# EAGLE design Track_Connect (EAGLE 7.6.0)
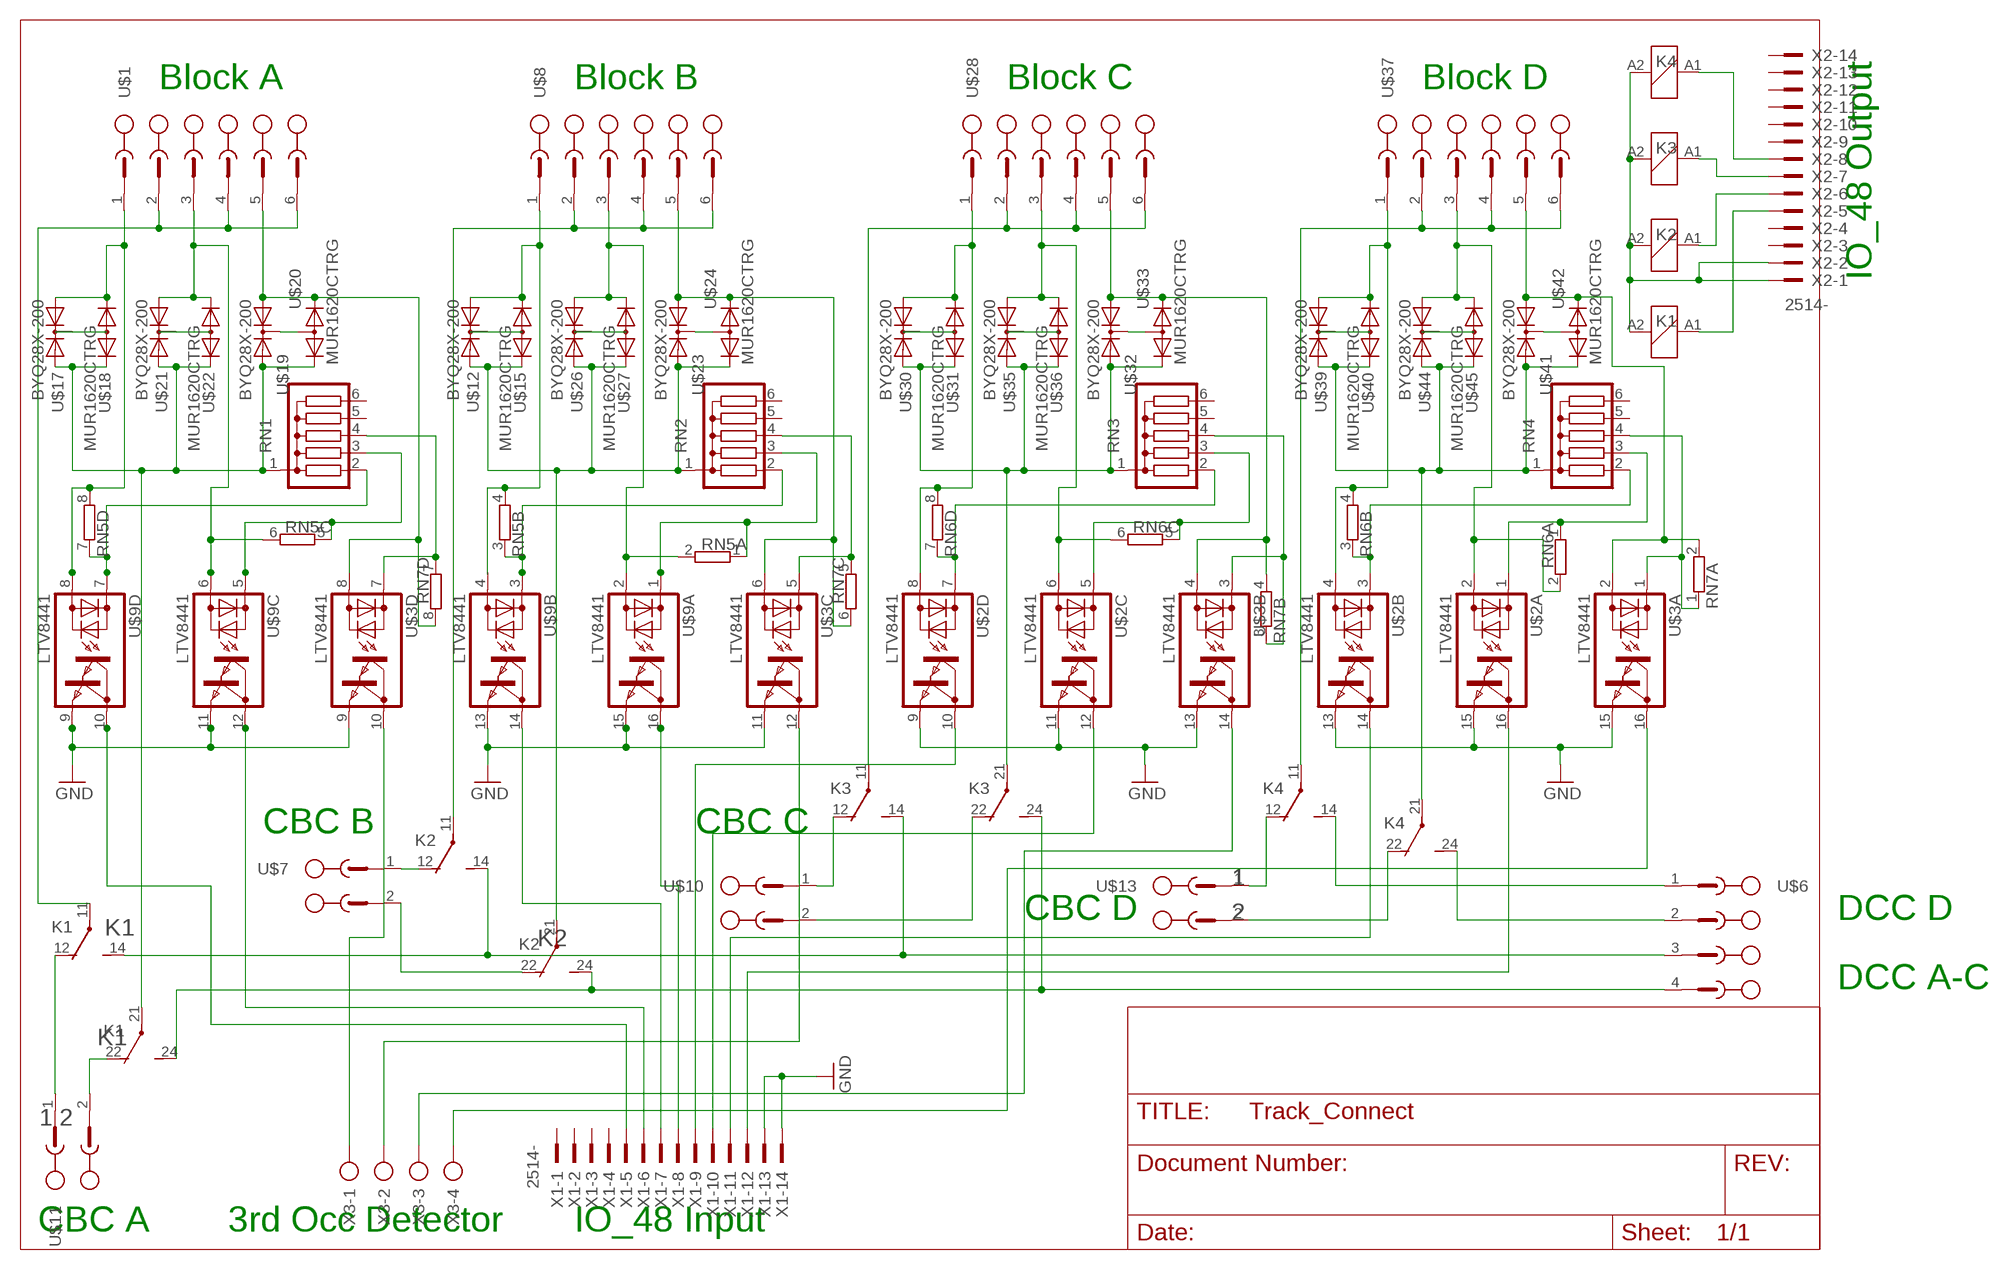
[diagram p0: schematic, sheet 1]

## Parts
K1  RT424012  [RT2C/O]
K2  RT424012  [RT2C/O]
K3  RT424012  [RT2C/O]
K4  RT424012  [RT2C/O]
RN1  G05R  [SIL6]
RN2  G05R  [SIL6]
RN3  G05R  [SIL6]
RN4  G05R  [SIL6]
RN5  E4R  [SIL8]
RN6  E4R  [SIL8]
RN7  E4R  [SIL8]
U$1  PT1_5_6-PVH-50  [PT1_5_6-PVH-50]
U$2  LTV8441  [DIL16]
U$3  LTV8441  [DIL16]
U$6  PT1_5_4-PVH-50  [PT1_5_4-PVH-50]
U$7  PT1_5_2-PVH-50  [PT1_5_2-PVH-50]
U$8  PT1_5_6-PVH-50  [PT1_5_6-PVH-50]
U$9  LTV8441  [DIL16]
U$10  PT1_5_2-PVH-50  [PT1_5_2-PVH-50]
U$11  PT1_5_2-PVH-50  [PT1_5_2-PVH-50]
U$12  BYQ28X-200  [TO220ABS]
U$13  PT1_5_2-PVH-50  [PT1_5_2-PVH-50]
U$15  MUR1620CTRG  [TO220ABS]
U$17  BYQ28X-200  [TO220ABS]
U$18  MUR1620CTRG  [TO220ABS]
U$19  BYQ28X-200  [TO220ABS]
U$20  MUR1620CTRG  [TO220ABS]
U$21  BYQ28X-200  [TO220ABS]
U$22  MUR1620CTRG  [TO220ABS]
U$23  BYQ28X-200  [TO220ABS]
U$24  MUR1620CTRG  [TO220ABS]
U$26  BYQ28X-200  [TO220ABS]
U$27  MUR1620CTRG  [TO220ABS]
U$28  PT1_5_6-PVH-50  [PT1_5_6-PVH-50]
U$30  BYQ28X-200  [TO220ABS]
U$31  MUR1620CTRG  [TO220ABS]
U$32  BYQ28X-200  [TO220ABS]
U$33  MUR1620CTRG  [TO220ABS]
U$35  BYQ28X-200  [TO220ABS]
U$36  MUR1620CTRG  [TO220ABS]
U$37  PT1_5_6-PVH-50  [PT1_5_6-PVH-50]
U$39  BYQ28X-200  [TO220ABS]
U$40  MUR1620CTRG  [TO220ABS]
U$41  BYQ28X-200  [TO220ABS]
U$42  MUR1620CTRG  [TO220ABS]
U$44  BYQ28X-200  [TO220ABS]
U$45  MUR1620CTRG  [TO220ABS]
X1  2514-  [PAK100/2500-14]
X2  2514-  [PAK100/2500-14]
X3  AK300/4  [AK300/4]

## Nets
GND: U$2.9(D:E) U$2.11(C:E) U$2.13(B:E) U$2.15(A:E) U$3.9(D:E) U$3.11(C:E) U$3.13(B:E) U$3.15(A:E) U$9.9(D:E) U$9.11(C:E) U$9.13(B:E) U$9.15(A:E) X1.13 X1.14
N$1: RN2.2 RN5.3 U$9.3(B:AC1)
N$2: RN1.3 RN5.5 U$9.5(C:AC1)
N$3 [Track]: K3.12(2:O) U$10.1(SK)
N$4: RN1.4 RN7.7 U$3.7(D:AC1)
N$5 [Track]: RN5.6 U$1.3(SK2) U$9.6(C:AC2) U$21.A1 U$22.A2(C2)
N$7 [Track]: U$21.C U$22.C(A)
N$8: RN2.3 RN5.1 U$9.1(A:AC1)
N$9: K1.21(3:P) RN1.1 U$17.A2 U$18.A1(C1) U$19.A2 U$20.A1(C1) U$21.A2 U$22.A1(C1)
N$12: K2.A1 X2.6
N$13 [Track]: K2.12(2:O) U$7.1(SK)
N$14 [Track]: K1.11(2:P) U$1.2(SK1) U$1.4(SK3) U$1.6(SK5)
N$15 [Track]: U$17.C U$18.C(A)
N$16 [Track]: K1.12(2:O) U$11.1(SK)
N$17 [Track]: K2.22(3:O) U$7.2(SK1)
N$18 [Track]: K1.22(3:O) U$11.2(SK1)
N$19: U$9.10(D:C1) X1.5
N$20 [Track]: RN7.2 U$3.2(A:AC2) U$37.5(SK4) U$41.A1 U$42.A2(C2)
N$21 [Track]: U$12.C U$15.C(A)
N$22: U$9.12(C:C1) X1.6
N$23 [Track]: RN5.8 U$1.1(SK) U$9.8(D:AC2) U$17.A1 U$18.A2(C2)
N$25 [Track]: U$19.C U$20.C(A)
N$26 [Track]: RN7.8 U$1.5(SK4) U$3.8(D:AC2) U$19.A1 U$20.A2(C2)
N$27 [Track]: U$23.C U$24.C(A)
N$28 [Track]: RN7.6 U$3.6(C:AC2) U$8.5(SK4) U$23.A1 U$24.A2(C2)
N$29: K2.21(3:P) RN2.1 U$12.A2 U$15.A1(C1) U$23.A2 U$24.A1(C1) U$26.A2 U$27.A1(C1)
N$30 [Track]: K2.11(2:P) U$8.2(SK1) U$8.4(SK3) U$8.6(SK5)
N$31 [Track]: U$26.C U$27.C(A)
N$32 [Track]: RN6.8 U$2.8(D:AC2) U$28.1(SK) U$30.A1 U$31.A2(C2)
N$33: RN2.4 RN7.5 U$3.5(C:AC1)
N$34: RN3.3 RN6.5 U$2.5(C:AC1)
N$35 [Track]: RN5.2 U$8.3(SK2) U$9.2(A:AC2) U$26.A1 U$27.A2(C2)
N$37 [Track]: RN5.4 U$8.1(SK) U$9.4(B:AC2) U$12.A1 U$15.A2(C2)
N$38: RN3.2 RN6.7 U$2.7(D:AC1)
N$39: RN1.2 RN5.7 U$9.7(D:AC1)
N$40: U$9.16(A:C1) X1.8
N$41: U$3.12(C:C1) X3.2
N$42: U$2.10(D:C1) X1.9
N$43 [Track]: K1.14(2:S) K2.14(2:S) K3.14(2:S) U$6.3(SK2)
N$44 [Track]: K1.24(3:S) K2.24(3:S) K3.24(3:S) U$6.4(SK3)
N$45: K1.A1 X2.5
N$46: K3.A1 X2.7
N$47 [Track]: U$30.C U$31.C(A)
N$49 [Track]: U$32.C U$33.C(A)
N$50 [Track]: RN7.4 U$3.4(B:AC2) U$28.5(SK4) U$32.A1 U$33.A2(C2)
N$51: K3.21(3:P) RN3.1 U$30.A2 U$31.A1(C1) U$32.A2 U$33.A1(C1) U$35.A2 U$36.A1(C1)
N$52 [Track]: K3.11(2:P) U$28.2(SK1) U$28.4(SK3) U$28.6(SK5)
N$53: U$2.12(C:C1) X1.10
N$54 [Track]: U$35.C U$36.C(A)
N$55 [Track]: RN6.6 U$2.6(C:AC2) U$28.3(SK2) U$35.A1 U$36.A2(C2)
N$56: RN3.4 RN7.3 U$3.3(B:AC1)
N$57: U$9.14(B:C1) X1.7
N$58: K1.A2 K2.A2 K3.A2 K4.A2 X2.1 X2.2
N$59: U$3.10(D:C1) X3.1
N$60 [Track]: K3.22(3:O) U$10.2(SK1)
N$62: RN4.2 RN6.3 U$2.3(B:AC1)
N$63: RN4.3 RN6.1 U$2.1(A:AC1)
N$64: U$2.14(B:C1) X1.11
N$65 [Track]: K4.12(2:O) U$13.1(SK)
N$67 [Track]: K4.11(2:P) U$37.2(SK1) U$37.4(SK3) U$37.6(SK5)
N$68 [Track]: U$39.C U$40.C(A)
N$69 [Track]: RN6.4 U$2.4(B:AC2) U$37.1(SK) U$39.A1 U$40.A2(C2)
N$70 [Track]: U$41.C U$42.C(A)
N$71: K4.A1 X2.8
N$73 [Track]: K4.21(3:P) RN4.1 U$39.A2 U$40.A1(C1) U$41.A2 U$42.A1(C1) U$44.A2 U$45.A1(C1)
N$75 [Track]: U$44.C U$45.C(A)
N$76: U$2.16(A:C1) X1.12
N$77: U$3.16(A:C1) X3.4
N$79 [Track]: K4.14(2:S) U$6.1(SK)
N$80 [Track]: K4.22(3:O) U$13.2(SK1)
N$81 [Track]: K4.24(3:S) U$6.2(SK1)
N$86: U$3.14(B:C1) X3.3
N$87 [Track]: RN6.2 U$2.2(A:AC2) U$37.3(SK2) U$44.A1 U$45.A2(C2)
N$88: RN4.4 RN7.1 U$3.1(A:AC1)
Unconnected: RN1.5 RN1.6 RN2.5 RN2.6 RN3.5 RN3.6 RN4.5 RN4.6 X1.1 X1.2 X1.3 X1.4 X2.3 X2.4 X2.9 X2.10 X2.11 X2.12 X2.13 X2.14

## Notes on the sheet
- Block A | Block B | Block C | Block D
- IO_48 Output
- CBC B | CBC C
- 1 | 1
- 2
- K1 | CBC D | DCC D
- K2
- DCC A-C
- K1
- 1 2
- CBC A | 3rd Occ Detector | IO_48 Input

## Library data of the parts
K1-K4 = relay:RT42?*: Power PCB Relay SCHRACK 2 pole 8 A, DC and AC-coil Source: http://www.schrack.com/.. 5842.pdf; MPN: RT424012; OC_FARNELL: 1629053; OC_NEWARK: 03P2426
RN1-RN4 = resistor-sil:G05R: SIL RESISTOR; OC_FARNELL: unknown; OC_NEWARK: unknown
RN5-RN7 = resistor-sil:E4R: SIL RESISTOR; OC_FARNELL: unknown; OC_NEWARK: unknown
U$1 U$8 U$28 U$37 = BDL-Boards:PT1_5_6-PVH-50
U$2 U$3 U$9 = optocoupler:LTV8441: Quad AC Optocoupler with Darlington Output
U$6 = BDL-Boards:PT1_5_4-PVH-50
U$7 U$11 = BDL-Board:PT1_5_2-PVH-50
U$10 U$13 = BDL-Boards:PT1_5_2-PVH-50
U$12 U$17 U$19 U$21 U$23 U$26 U$30 U$32 U$35 U$39 U$41 U$44 = diode:BYQ28X-200: Fast Recovery Diode Pair Common Cathode 10 Amps
U$15 U$18 U$20 U$22 U$24 U$27 U$31 U$33 U$36 U$40 U$42 U$45 = diode:MUR1620CTRG: Fast Recovery Diode Halfbridge 16 Amps
X1 X2 = con-3m:2514-: 3M (TM) Pak 100 4-Wall Header Source: 3M; OC_FARNELL: unknown; OC_NEWARK: unknown
X3 = con-ptr500:AK300/4: CONNECTOR; OC_FARNELL: unknown; OC_NEWARK: unknown

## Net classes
0 default: width 0.762 mm, drill 0.508 mm, clearance 0.381 mm
1 GND: width 0.762 mm, drill 0.508 mm, clearance 0.381 mm
2 VCC1: width 1.27 mm, drill 0.508 mm, clearance 0.381 mm
3 VCC2: width 0.762 mm, drill 0.508 mm, clearance 0.381 mm
4 Track: width 2.032 mm, drill 0.508 mm, clearance 0.381 mm

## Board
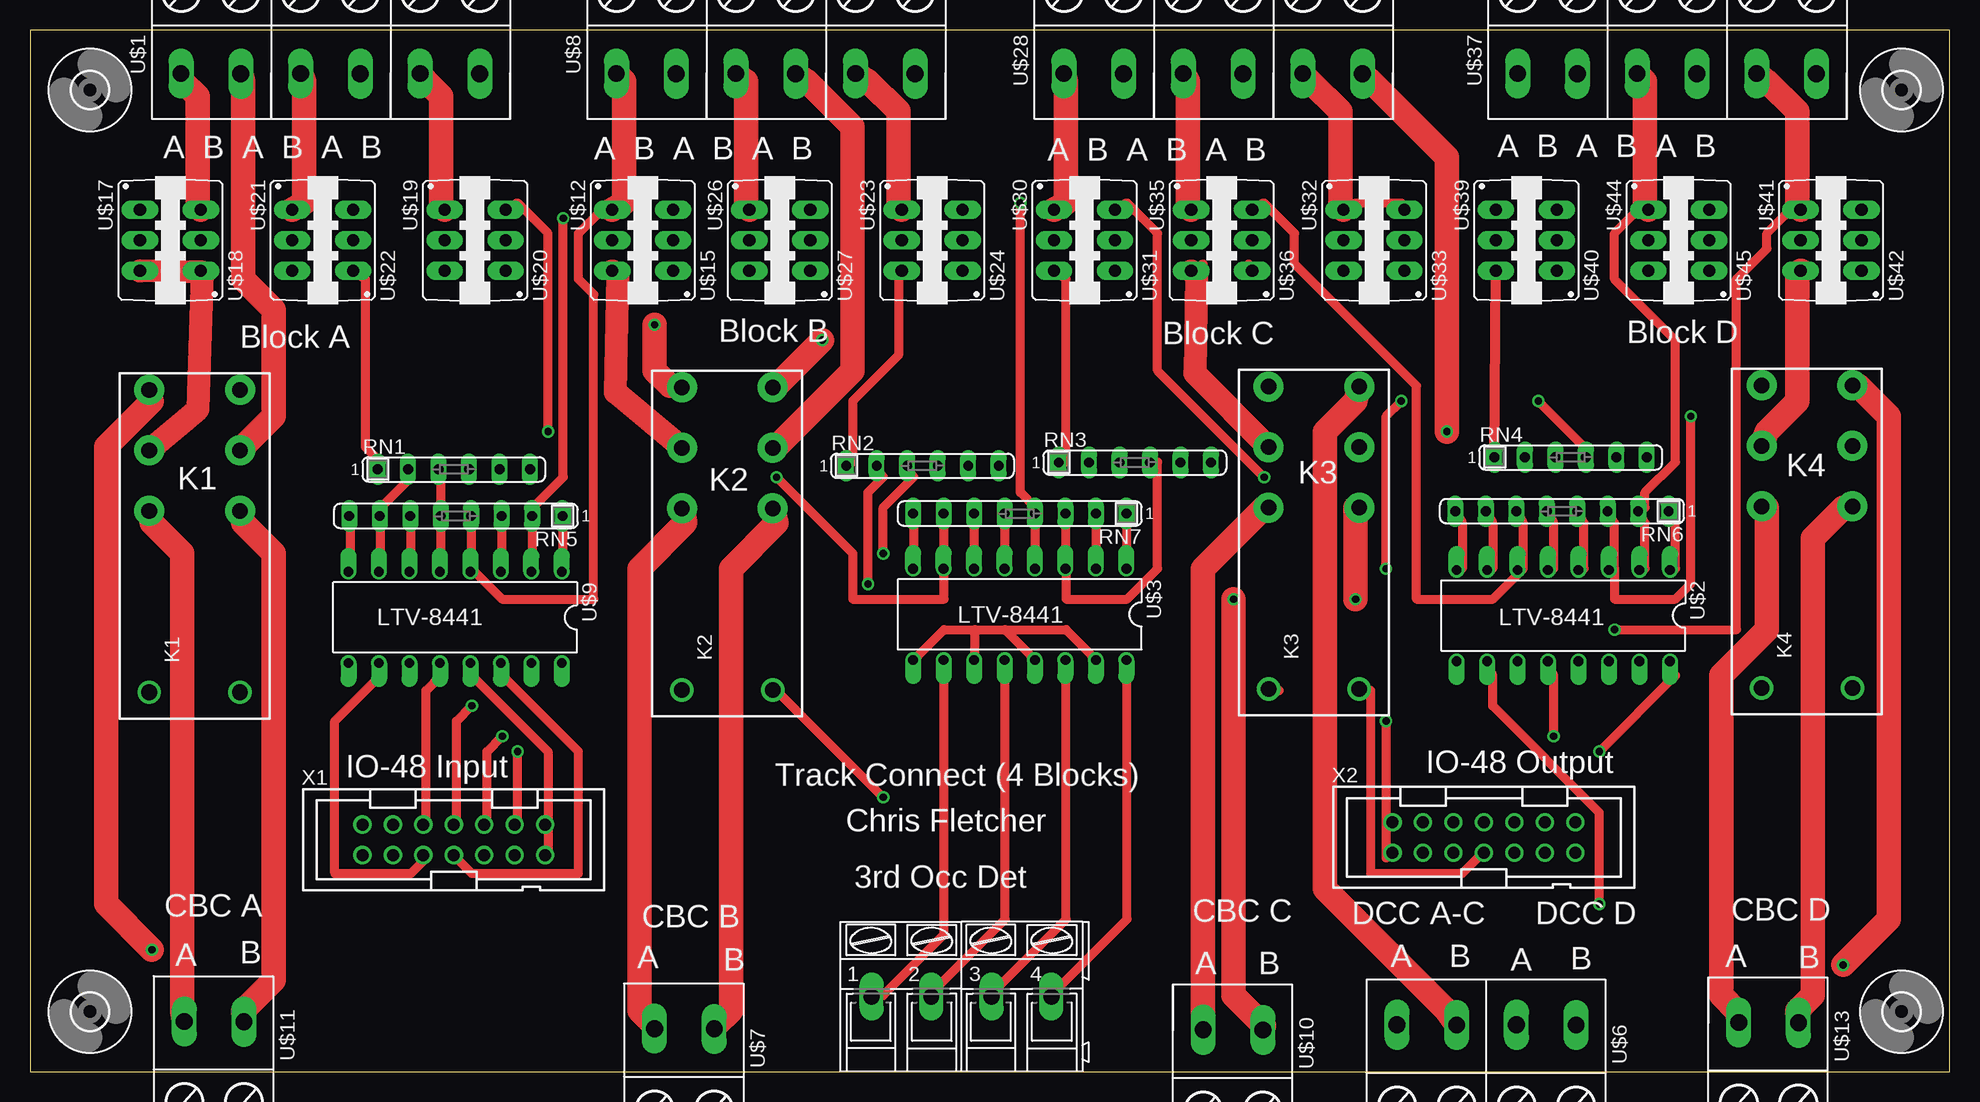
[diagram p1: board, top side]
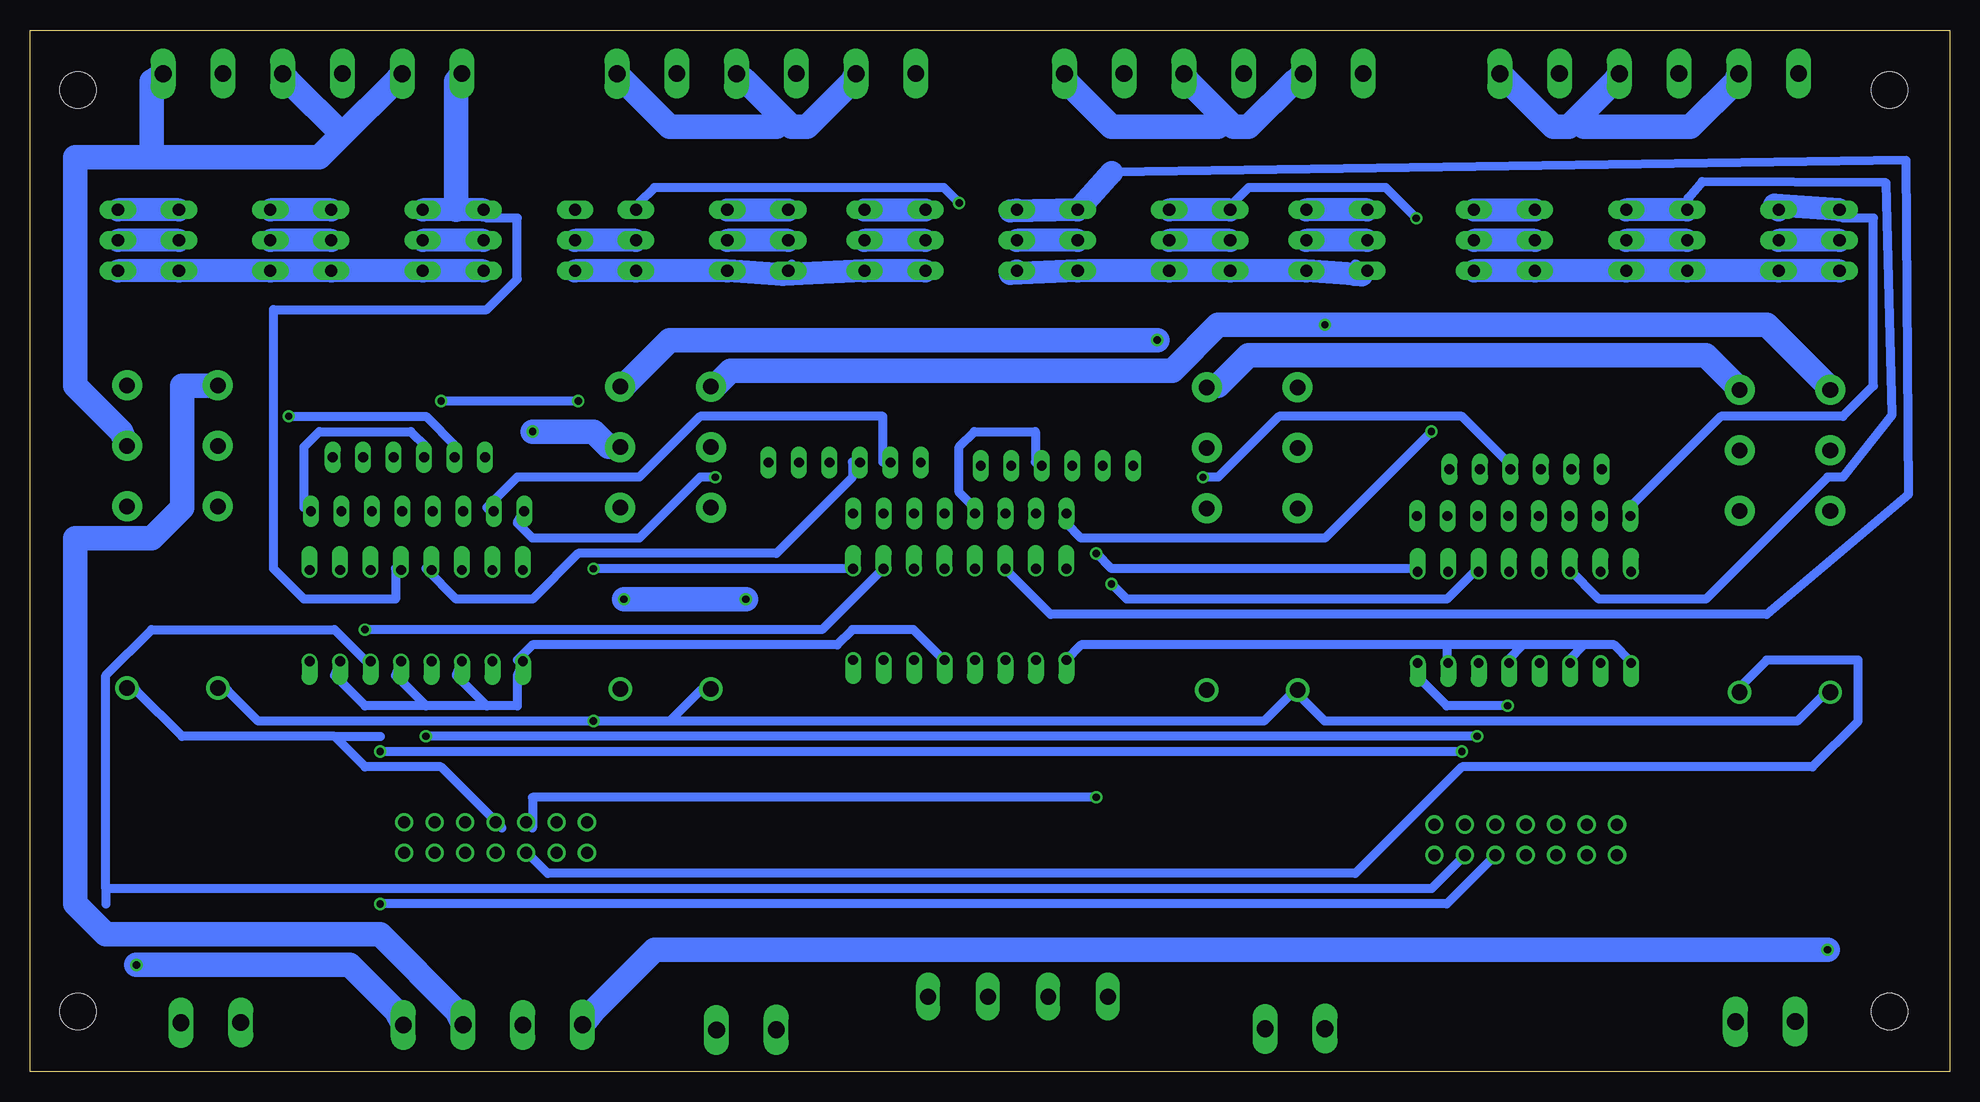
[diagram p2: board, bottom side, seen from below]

Size 160 x 86.8 mm. Coordinates in mm from the lower left corner, seen from the top.
Outline: 0,0 160,0 160,86.8 0,86.8 0,0
Copper layers (1*16): Top 0.035mm / dielectric 1.5mm / Bottom 0.035mm
Design rules "default": minimum track width 10mil, minimum drill 24mil, track to track 8mil, track to pad 8mil, pad to pad 8mil, via to via 8mil, smd to smd 8mil, copper to edge 40mil, drill to drill 8mil, minimum pad ring 10mil, minimum via ring 8mil, stop-mask expansion 4mil, vias tented up to drill 0mil, thermal gap 10mil

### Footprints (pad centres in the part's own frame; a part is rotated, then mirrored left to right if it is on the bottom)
3,0 = hole 3: 0,0
RT2C/O = drill 1.3 pad 2.5: 11 7.56,-3.68; 12 2.52,-3.68; 14 12.6,-3.68; 21 7.56,3.88; 22 2.52,3.88; 24 12.6,3.88 | drill 1.3: A1 -12.6,-3.68; A2 -12.6,3.88
SIL6 = drill 0.813 long: 1 -6.35,0; 2 -3.81,0; 3 -1.27,0; 4 1.27,0; 5 3.81,0; 6 6.35,0
SIL8 = drill 0.813 long: 1 -8.89,0; 2 -6.35,0; 3 -3.81,0; 4 -1.27,0; 5 1.27,0; 6 3.81,0; 7 6.35,0; 8 8.89,0
PT1_5_6-PVH-50 = drill 1.397 long: 1 17.157,2.42; 2 12.181,2.44; 3 7.197,2.42; 4 2.221,2.44; 5 -2.763,2.42; 6 -7.739,2.44
DIL16 = drill 0.813 offset: 1 -8.89,-3.81; 2 -6.35,-3.81; 3 -3.81,-3.81; 4 -1.27,-3.81; 5 1.27,-3.81; 6 3.81,-3.81; 7 6.35,-3.81; 8 8.89,-3.81; 9 8.89,3.81; 10 6.35,3.81; 11 3.81,3.81; 12 1.27,3.81; 13 -1.27,3.81; 14 -3.81,3.81; 15 -6.35,3.81; 16 -8.89,3.81
PT1_5_4-PVH-50 = drill 1.397 long: 1 4.457,6.23; 2 -0.519,6.25; 3 -5.503,6.23; 4 -10.479,6.25
PT1_5_2-PVH-50 = drill 1.397 long: 1 1.917,2.42; 2 -3.059,2.44
TO220ABS = drill 1.016 long: A1 -2.54,-2.54; A2 2.54,-2.54; C 0,-2.54
PAK100/2500-14 = drill 1 pad 1.422: 1 -7.62,-1.27; 2 -7.62,1.27; 3 -5.08,-1.27; 4 -5.08,1.27; 5 -2.54,-1.27; 6 -2.54,1.27; 7 0,-1.27; 8 0,1.27; 9 2.54,-1.27; 10 2.54,1.27; 11 5.08,-1.27; 12 5.08,1.27; 13 7.62,-1.27; 14 7.62,1.27
AK300/4 = drill 1.321 long: 1 -7.493,0; 2 -2.515,0; 3 2.515,0; 4 7.493,0

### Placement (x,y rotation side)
E$1  [3,0]  5,81.8 0 top
E$2  [3,0]  156,81.8 0 top
E$3  [3,0]  5,5 0 top
E$4  [3,0]  156,5 0 top
K1  13.82,44.21 90 top
K2  58.22,44.41 90 top
K3  107.12,44.48 90 top
K4  148.22,44.58 90 top
RN1  35.33,50.19 0 top
RN2  74.39,50.49 0 top
RN3  92.09,50.76 0 top
RN4  128.42,51.19 0 top
RN5  35.5,46.3 180 top
RN6  127.7,46.7 180 top
RN7  82.5,46.5 180 top
U$1  29.75,85.59 180 top
U$2  127.8,38 180 top
U$3  82.5,38.1 180 top
U$6  124.42,-2.34 0 top
U$7  55.12,1.14 0 top
U$8  66.04,85.59 180 top
U$9  35.44,37.85 180 top
U$10  100.86,1.05 0 top
U$11  15.92,1.74 0 top
U$12  51.07,69.27 270 top
U$13  145.49,1.65 0 top
U$15  51.07,69.27 90 top
U$17  11.7,69.27 270 top
U$18  11.7,69.27 90 top
U$19  37.1,69.27 270 top
U$20  37.1,69.27 90 top
U$21  24.4,69.27 270 top
U$22  24.4,69.27 90 top
U$23  75.2,69.27 270 top
U$24  75.2,69.27 90 top
U$26  62.5,69.27 270 top
U$27  62.5,69.27 90 top
U$28  103.33,85.59 180 top
U$30  87.9,69.27 270 top
U$31  87.9,69.27 90 top
U$32  112.03,69.27 270 top
U$33  112.03,69.27 90 top
U$35  99.33,69.27 270 top
U$36  99.33,69.27 90 top
U$37  141.16,85.59 180 top
U$39  124.73,69.27 270 top
U$40  124.73,69.27 90 top
U$41  150.13,69.27 270 top
U$42  150.13,69.27 90 top
U$44  137.43,69.27 270 top
U$45  137.43,69.27 90 top
X1  35.33,19.32 0 top
X2  121.2,19.52 0 top
X3  77.64,6.25 0 top

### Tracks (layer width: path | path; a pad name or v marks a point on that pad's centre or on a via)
GND
  Top 0.762: 78.74,36.83 76.2,36.83 73.66,34.29 U$3.9 | 78.74,36.83 78.74,34.29 U$3.11 | 81.28,36.83 83.82,34.29 U$3.13 | 78.74,36.83 81.28,36.83 | 81.28,36.83 86.36,36.83 88.9,34.29 U$3.15 | U$9.13 36.83,33.02 43.18,26.67 43.18,20.32 | 43.18,20.32 43.18,17.78 X1.13 | 43.18,20.32 X1.14
  Bottom 0.762: 121.92,30.48 119.38,30.48 119.38,33.02 U$2.9 119.38,34.29 118.11,35.56 92.71,35.56 91.44,36.83 86.36,36.83 83.82,34.29 U$3.13 | 121.92,30.48 124.46,33.02 U$2.11 | 127,30.48 129.54,33.02 U$2.13 | 121.92,30.48 127,30.48 | 127,30.48 132.08,30.48 134.62,33.02 U$2.15 | 30.48,35.56 27.94,35.56 26.67,34.29 U$9.9 | 30.48,35.56 31.75,34.29 U$9.11 | 35.56,35.56 36.83,34.29 U$9.13 | 30.48,35.56 35.56,35.56 | 35.56,35.56 41.91,35.56 | 41.91,35.56 72.39,35.56 73.66,34.29 U$3.9 | 41.91,35.56 41.91,34.29 U$9.15
N$1  (via drill 0.61)
  Top 0.762: U$9.3 39.37,41.91 39.37,45.72 RN5.3 | v69.85,40.64 69.85,48.26 71.12,49.53 RN2.2
  Bottom 0.762: v69.85,40.64 68.58,39.37 41.91,39.37 39.37,41.91 U$9.3
N$2
  Top 0.762: U$9.5 34.29,41.91 34.29,45.72 RN5.5 34.29,46.99 34.29,49.53 RN1.3
N$3  (via drill 0.61)
  Top 2.032: v100.33,39.37 100.33,6.35 102.87,3.81 U$10.1 | v110.49,39.37 110.49,46.99 K3.12
  Bottom 2.032: v100.33,39.37 v110.49,39.37
N$4  (via drill 0.61)
  Top 0.762: 76.2,41.91 76.2,45.72 RN7.7 | v62.23,49.53 68.58,43.18 68.58,39.37 76.2,39.37 76.2,41.91 | 76.2,41.91 U$3.7
  Bottom 0.762: v62.23,49.53 60.96,49.53 55.88,54.61 40.64,54.61 36.83,50.8 RN1.4
N$5
  Top 0.762: U$9.6 31.75,41.91 31.75,45.72 RN5.6
  Top 2.032: U$1.3 22.86,82.55 22.86,72.39 U$21.A1
  Bottom 0.762: U$9.6 31.75,41.91 29.21,39.37 20.32,39.37 10.16,49.53 8.89,49.53 4.78,54.74 5.28,74.06 20.62,74.16 21.79,72.79 U$21.A1
  Bottom 1.93: U$21.A1 U$22.A2
N$7
  Bottom 1.93: U$21.C U$22.C
N$8  (via drill 0.61)
  Top 0.762: U$9.1 44.45,41.91 44.45,45.72 RN5.1 | v71.12,43.18 71.12,46.99 73.66,49.53 RN2.3
  Bottom 0.762: v71.12,43.18 69.85,41.91 44.45,41.91 U$9.1
N$9
  Top 0.762: RN1.1 29.21,50.8 27.94,52.07 27.94,66.04 U$22.A1
  Top 1.93: U$17.A2 14.4,66.6 14,55.2 K1.21
  Bottom 1.93: U$17.A2 U$18.A1 U$21.A2 U$22.A1 U$19.A2 U$20.A1
N$12  (via drill 0.61)
  Top 0.762: v71.12,22.86 62.23,31.75 K2.A1
  Bottom 0.762: v71.12,22.86 118.11,22.86 118.11,20.32 X2.6
N$13
  Top 2.032: U$7.1 57.15,3.81 58.42,5.08 58.42,41.91 62.23,45.72 K2.12
N$14
  Top 2.032: K1.11 17.78,52.07 20.32,54.61 20.32,63.5 17.78,66.04 17.78,82.55 U$1.2
  Bottom 2.032: 31.11,79.38 31.75,78.74 33.02,78.74 36.83,82.55 U$1.6 | 31.11,79.38 27.94,82.55 U$1.4 | U$1.2 17.78,82.55 21.59,78.74 30.48,78.74 31.11,79.38
N$15
  Bottom 1.93: U$17.C U$18.C
N$16
  Top 2.032: U$11.1 17.78,5.08 20.32,7.62 20.32,43.18 17.78,45.72 K1.12
N$17
  Top 2.032: U$7.2 52.07,3.81 50.8,5.08 50.8,41.91 54.61,45.72 K2.22
N$18
  Top 2.032: U$11.2 12.7,5.08 12.7,43.18 10.16,45.72 K1.22
N$19
  Top 0.762: U$9.10 29.21,33.02 25.4,29.21 25.4,16.51 31.75,16.51 33.02,17.78 X1.5
N$20  (via drill 0.61)
  Top 0.762: U$3.2 88.9,41.91 88.9,45.72 RN7.2 | v132.08,36.83 142.24,36.83 142.24,66.04 144.78,68.58 144.78,69.85 147.32,72.39
  Top 2.032: U$37.5 144.78,82.55 147.32,80.01 147.32,72.39 U$41.A1
  Bottom 0.762: v132.08,36.83 93.98,36.83 88.9,41.91 U$3.2
  Bottom 1.93: U$41.A1 U$42.A2
N$21
  Bottom 1.93: U$12.C U$15.C
N$22
  Top 0.762: U$9.12 34.29,33.02 33.02,31.75 33.02,20.32 X1.6
N$23
  Top 0.762: U$9.8 26.67,41.91 26.67,45.72 RN5.8
  Top 2.032: U$1.1 12.7,82.55 13.97,81.28 13.97,72.39 U$18.A2
  Bottom 0.762: RN5.8 26.67,46.99 19.05,54.61 8.89,54.61 6.35,57.15 6.35,71.12 8.89,71.12 U$17.A1
  Bottom 1.93: U$17.A1 14.6,72.2 U$18.A2
N$25
  Bottom 1.93: U$19.C U$20.C
N$26  (via drill 0.61)
  Top 0.762: U$3.8 73.66,41.91 73.66,45.72 RN7.8 | v43.18,53.34 43.18,69.85 40.64,72.39 U$20.A2
  Top 2.032: U$1.5 33.02,82.55 34.29,81.28 34.29,72.39 U$19.A1
  Bottom 0.762: v43.18,53.34 52.07,44.45 72.39,44.45 73.66,45.72 RN7.8
  Bottom 1.93: U$20.A2 U$19.A1
N$27
  Bottom 1.93: U$23.C U$24.C
N$28
  Top 0.762: U$3.6 78.74,41.91 78.74,45.72 RN7.6
  Top 2.032: U$8.5 69.85,82.55 72.39,80.01 72.39,72.39 U$23.A1
  Bottom 0.762: U$3.6 78.74,41.91 74.93,38.1 15.24,38.1 3.41,48.13 3.61,75.93 69.85,74.93 72.39,72.39 U$23.A1
  Bottom 1.93: U$23.A1 78.3,71.7 U$24.A2 | 69.85,74.93 72.7,71.8
N$29
  Top 0.762: RN2.1 68.58,50.8 68.58,55.88 72.39,59.69 72.39,66.04 U$23.A2
  Top 1.93: K2.21 48.8,56.6 49,66.4 U$12.A2
  Bottom 0.762: U$12.A2 49.53,67.31 49.59,66.45
  Bottom 1.93: 49,66.4 49.59,66.45 U$15.A1 U$26.A2 U$27.A1 U$23.A2 78.3,66.5 U$24.A1
N$30
  Top 2.032: K2.11 62.23,52.07 68.58,58.42 68.58,78.74 64.77,82.55 U$8.4
  Bottom 2.032: 60.33,79.38 63.5,82.55 U$8.4 | 60.33,79.38 59.69,78.74 58.42,78.74 54.61,82.55 U$8.2 | U$8.6 73.66,82.55 69.85,78.74 60.96,78.74 60.33,79.38
N$31
  Bottom 1.93: U$26.C U$27.C
N$32  (via drill 0.61)
  Top 0.762: RN6.8 119.38,45.72 119.38,41.91 U$2.8 | v102.87,49.53 93.98,58.42 93.98,69.85 91.44,72.39 U$31.A2
  Top 2.032: U$28.1 86.36,82.55 86.36,72.39 U$30.A1
  Bottom 0.762: v102.87,49.53 104.14,49.53 109.22,44.45 118.11,44.45 119.38,45.72 RN6.8
  Bottom 1.93: U$31.A2 U$30.A1
N$33
  Top 0.762: U$3.5 81.28,41.91 81.28,45.72 RN7.5
  Bottom 0.762: RN2.4 76.2,50.8 76.2,53.34 81.28,53.34 82.55,52.07 82.55,48.26 81.28,46.99 RN7.5
N$34
  Top 0.762: RN6.5 127,45.72 127,41.91 U$2.5
  Bottom 0.762: RN3.3 91.44,50.8 91.44,49.53 97.79,43.18 114.3,43.18 118.11,39.37 124.46,39.37 127,41.91 U$2.5
N$35  (via drill 0.61)
  Top 0.762: U$9.2 41.91,41.91 41.91,45.72 RN5.2 41.91,46.99 44.45,49.53 v44.45,71.12
  Top 2.032: U$8.3 59.69,82.55 59.69,72.39 U$26.A1
  Bottom 0.762: v44.45,71.12 46.99,73.66 58.42,73.66 59.69,72.39 U$26.A1
  Bottom 1.93: U$26.A1 U$27.A2
N$37
  Top 0.762: 36.83,41.91 36.83,45.72 RN5.4 | 36.83,41.91 39.37,39.37 46.99,39.37 46.99,64.77 45.72,66.04 45.72,69.85 48.26,72.39 U$12.A1 | U$9.4 36.83,41.91
  Top 2.032: U$8.1 49.53,82.55 49.53,72.39 U$12.A1
  Bottom 1.93: U$12.A1 U$15.A2
N$38
  Top 0.762: RN6.7 121.92,45.72 121.92,41.91 U$2.7
  Bottom 0.762: RN3.2 88.9,50.8 88.9,54.61 104.14,54.61 109.22,49.53 119.38,49.53 121.92,46.99 RN6.7
N$39
  Top 0.762: U$9.7 29.21,41.91 29.21,45.72 RN5.7 29.21,46.99 31.75,49.53 RN1.2
N$40  (via drill 0.61)
  Top 0.762: v36.83,30.48 35.56,29.21 35.56,20.32 X1.8
  Bottom 0.762: v36.83,30.48 41.91,30.48 44.45,33.02 U$9.16
N$41
  Top 0.762: U$3.12 81.28,34.29 81.28,12.7 74.93,6.35 X3.2
N$42  (via drill 0.61)
  Top 0.762: v130.81,13.97 130.81,21.59 121.92,30.48 121.92,33.02 U$2.10
  Bottom 0.762: v130.81,13.97 41.91,13.97 38.1,17.78 X1.9
N$43  (via drill 0.61)
  Top 2.032: K3.14 110.49,55.88 107.95,53.34 107.95,15.24 118.11,5.08 U$6.3 | v66.04,60.96 62.23,57.15 K2.14
  Bottom 2.032: K1.14 17.78,57.15 20.32,59.69 58.42,59.69 60.96,57.15 K2.14 | v66.04,60.96 106.68,60.96 110.49,57.15 K3.14
N$44  (via drill 0.61)
  Top 2.032: v10.16,10.16 6.35,13.97 6.35,52.07 10.16,55.88 K1.24 | v52.07,62.23 52.07,58.42 53.34,57.15 K2.24
  Bottom 2.032: v10.16,10.16 107.95,10.16 113.03,5.08 U$6.4 | K1.24 10.16,57.15 15.24,62.23 v52.07,62.23 60.96,62.23 64.77,58.42 101.6,58.42 102.87,57.15 K3.24
N$45
  Bottom 0.762: K1.A1 17.78,31.75 15.24,34.29 7.62,34.29 7.62,29.21 11.43,25.4 40.64,25.4 49.53,16.51 116.84,16.51 118.11,17.78 X2.5
N$46
  Top 0.762: 110.49,31.75 K3.A1 111.76,31.75 111.76,16.51 119.38,16.51 120.65,17.78 X2.7
N$47
  Bottom 1.93: U$30.C U$31.C
N$49
  Bottom 1.93: U$32.C U$33.C
N$50  (via drill 0.61)
  Top 0.762: U$3.4 83.82,41.91 83.82,45.72 RN7.4 83.82,46.99 82.55,48.26 v82.55,72.39 | U$33.A2 114.3,72.39 110.49,72.39 U$32.A1
  Top 2.032: U$28.5 106.68,82.55 109.22,80.01 109.22,72.39 U$32.A1
  Bottom 0.762: v82.55,72.39 83.82,73.66 107.95,73.66 109.22,72.39 U$32.A1
N$51
  Top 0.762: U$35.A2 97.79,67.31 | U$36.A1 101.6,67.31 | RN3.1 86.36,50.8 86.36,66.04 U$30.A2
  Top 1.93: K3.21 97.1,58.2 97.24,66.42 U$35.A2
  Bottom 0.762: 96.48,66.45 96.52,67.31 U$35.A2
  Bottom 1.93: U$33.A1 U$32.A2 U$36.A1 97.24,66.42 96.48,66.45 U$31.A1 U$30.A2
N$52  (via drill 0.61)
  Top 2.032: v118.11,53.34 118.11,76.2 111.76,82.55 U$28.6
  Bottom 2.032: 97.16,79.38 100.33,82.55 U$28.4 | 97.16,79.38 96.52,78.74 95.25,78.74 91.44,82.55 U$28.2 | U$28.6 110.49,82.55 106.68,78.74 97.79,78.74 97.16,79.38 | v118.11,53.34 113.03,53.34 111.76,52.07 K3.11
N$53  (via drill 0.61)
  Top 0.762: v127,27.94 127,33.02 U$2.12 | v39.37,27.94 38.1,26.67 38.1,20.32 X1.10
  Bottom 0.762: v39.37,27.94 v127,27.94
N$54
  Bottom 1.93: U$35.C U$36.C
N$55
  Top 0.762: 124.46,41.91 124.46,45.72 RN6.6 | 124.46,41.91 121.92,39.37 115.57,39.37 115.57,57.15 105.41,67.31 105.41,69.85 102.87,72.39 U$36.A2 | 124.46,41.91 U$2.6
  Top 2.032: U$28.3 96.52,82.55 96.52,72.39 U$35.A1
  Bottom 1.93: U$36.A2 U$35.A1
N$56
  Top 0.762: 86.36,41.91 86.36,45.72 RN7.3 | 86.36,41.91 86.36,39.37 91.44,39.37 93.98,41.91 93.98,50.8 RN3.4 | U$3.3 86.36,41.91
N$57
  Top 0.762: U$9.14 39.37,33.02 45.72,26.67 45.72,16.51 36.83,16.51 35.56,17.78 X1.7
N$58  (via drill 0.61)
  Top 0.762: K3.A2 104.14,31.75 | 113.03,20.32 113.03,17.78 X2.1 | v113.03,29.21 113.03,20.32 | 113.03,20.32 X2.2
  Bottom 0.762: 54.61,31.75 52.07,29.21 12.7,29.21 10.16,31.75 K1.A2 | 106.68,29.21 v113.03,29.21 140.97,29.21 143.51,31.75 K4.A2 | 106.68,29.21 104.14,31.75 K3.A2 | 54.61,31.75 57.15,29.21 106.68,29.21 | 54.61,31.75 K2.A2
N$59
  Top 0.762: U$3.10 76.2,34.29 76.2,11.43 71.12,6.35 X3.1
N$60
  Top 2.032: U$10.2 97.79,3.81 97.79,41.91 102.87,46.99 K3.22
N$62  (via drill 0.61)
  Top 0.762: 132.08,41.91 132.08,45.72 RN6.3 | v138.43,54.61 138.43,40.64 137.16,39.37 132.08,39.37 132.08,41.91 | U$2.3 132.08,41.91
  Bottom 0.762: v138.43,54.61 127,54.61 124.46,52.07 RN4.2
N$63
  Top 0.762: RN6.1 137.16,45.72 137.16,41.91 U$2.1
  Bottom 0.762: RN4.3 127,52.07 128.27,53.34 135.89,53.34 137.16,52.07 137.16,46.99 RN6.1
N$64
  Bottom 0.762: 153.67,15.24 153.67,33.02 149.86,36.83 134.62,36.83 132.08,34.29 U$2.14 | 153.67,15.24 153.67,13.97 | 153.67,15.24 43.18,15.24 40.64,17.78 X1.11
N$65
  Top 2.032: U$13.1 147.32,5.08 148.59,6.35 148.59,44.45 151.13,46.99 K4.12
N$67
  Bottom 2.032: K4.11 152.4,53.34 156.21,57.15 156.21,76.2 149.86,76.2 | 133.99,78.11 135.89,76.2 149.86,76.2 | 133.99,78.11 129.54,82.55 U$37.2 | U$37.4 138.43,82.55 133.99,78.11 | 149.86,76.2 149.86,82.55 U$37.6
N$68
  Bottom 1.93: U$39.C U$40.C
N$69
  Top 0.762: RN6.4 129.54,45.72 129.54,41.91 U$2.4
  Bottom 0.762: U$2.4 129.54,41.91 129.54,39.37 137.16,39.37 139.7,41.91 139.7,63.5 121.92,63.5 119.38,66.04 119.38,71.12 121.92,71.12 U$39.A1
  Bottom 1.93: U$39.A1 124.46,71.81 U$40.A2
  Bottom 2.032: U$37.1 124.46,82.55 124.46,71.81
N$70
  Bottom 1.93: U$41.C U$42.C
N$71
  Bottom 0.762: 134.62,27.94 130.81,27.94 | 134.62,27.94 147.32,27.94 151.13,31.75 K4.A1 | 134.62,27.94 132.08,25.4 125.73,25.4 120.65,20.32 X2.8
N$73
  Top 0.813: RN4.1 U$39.A2
  Top 2.032: K4.21 144.78,53.34 147.32,55.88 147.32,66.04 U$41.A2
  Bottom 1.93: U$42.A1 U$41.A2 U$45.A1 U$44.A2 U$40.A1 U$39.A2
N$75
  Bottom 1.93: U$44.C U$45.C
N$76  (via drill 0.61)
  Top 0.762: v130.81,26.67 137.16,33.02 U$2.16 | v40.64,26.67 40.64,20.32 X1.12
  Bottom 0.762: v40.64,26.67 v130.81,26.67
N$77
  Top 0.762: U$3.16 91.44,34.29 91.44,12.7 85.09,6.35 X3.4
N$79  (via drill 0.61)
  Top 2.032: v151.13,8.89 154.94,12.7 154.94,54.61 152.4,57.15 K4.14
  Bottom 2.032: v151.13,8.89 133.35,8.89 129.54,5.08 U$6.1
N$80
  Top 2.032: U$13.2 142.24,5.08 140.97,6.35 140.97,33.02 144.78,36.83 144.78,46.99 K4.22
N$81
  Bottom 2.032: U$6.2 124.46,5.08 130.81,11.43 153.67,11.43 156.21,13.97 156.21,44.45 149.86,44.45 147.32,46.99 147.32,57.15 144.78,57.15 K4.24
N$86
  Top 0.762: U$3.14 86.36,34.29 86.36,12.7 80.01,6.35 X3.3
N$87
  Top 0.762: U$2.2 134.62,41.91 134.62,45.72 RN6.2 134.62,46.99 134.62,48.26 137.16,50.8 137.16,60.96 132.08,66.04 132.08,69.85 134.62,72.39
  Top 2.032: U$37.3 134.62,82.55 134.62,72.39 U$44.A1
  Bottom 1.93: U$44.A1 U$45.A2
N$88  (via drill 0.61)
  Top 0.762: U$3.1 91.44,41.91 91.44,45.72 RN7.1 | v125.73,55.88 129.54,52.07 RN4.4 | v114.3,55.88 113.03,54.61 v113.03,41.91
  Bottom 0.762: v114.3,55.88 v125.73,55.88 | U$3.1 v113.03,41.91

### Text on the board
tPlace: A B A B A B | A B A B A B | A B A B A B | A B A B A B | Block B | Block C | Block D | Block A | K4 | K3 | K1 | K2 | LTV-8441 | LTV-8441 | LTV-8441 | IO-48 Output | IO-48 Input | Track Connect (4 Blocks) | Chris Fletcher | 3rd Occ Det | CBC C | DCC A-C | DCC D | CBC D | CBC A | CBC B | A | B | A | A | B | A | B | B | A | B | A | B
